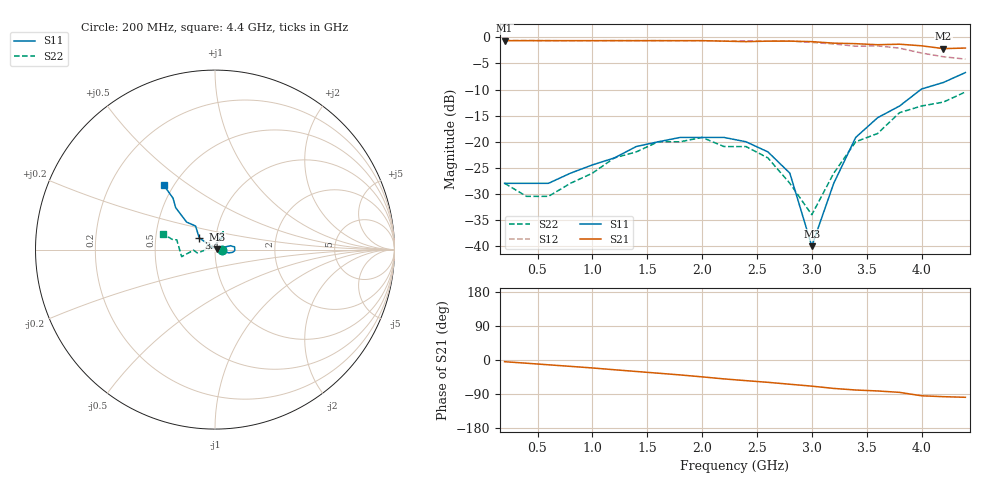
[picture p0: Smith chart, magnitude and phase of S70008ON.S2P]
!  MGS-70008 S PARAMETERS
!  "on" port  LAST UPDATED 07-22-92
# ghz s ma r 50
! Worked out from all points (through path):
!   22 points, 200 MHz to 4.4 GHz, reference 50 ohm
!   highest |S21| = -0.63 dB at 200 MHz (marker M1); lowest = -2.2 dB at 4.2 GHz (marker M2)
!   group delay of S21, straight-line fit = 64.8 ps
!   lowest |S11| = -40.0 dB at 3 GHz (marker M3), VSWR 1.02, Z = 51 + j0.131 ohm
!   |S11| at or under -10 dB: start of sweep to 3.994 GHz
!   |S22| runs from -34.0 to -10.5 dB; largest |S21 - S12| = 0.18
!   S11 on the Smith chart (normalised r, x): 200 MHz: 1.08, -0.01; 3.4 GHz: 0.83, +0.11; 4.4 GHz: 0.44, +0.40
0.2  0.04 -6.2  0.93 -4.5  0.934 -4.4  0.04 -2.5
0.4  0.04 0.3  0.93 -8.5  0.934 -8.3  0.03 10.6
0.6  0.04 7.6  0.93 -12.7  0.93 -12.4  0.03 30.7
0.8  0.05 13.6  0.93 -16.8  0.927 -16.3  0.04 52.8
1  0.06 14.7  0.93 -21.0  0.927 -20.4  0.05 63.0
1.2  0.07 14.5  0.93 -25.7  0.931 -24.5  0.07 67.1
1.4  0.09 14.0  0.93 -30.3  0.93 -28.7  0.08 69.1
1.6  0.1 10.2  0.93 -34.8  0.93 -32.9  0.1 69.2
1.8  0.11 8.1  0.93 -39.4  0.928 -37.6  0.1 66.6
2  0.11 1.4  0.93 -44.5  0.928 -41.8  0.11 65.2
2.2  0.11 -3.2  0.92 -49.9  0.922 -46.8  0.09 62.2
2.4  0.1 -8.5  0.91 -54.5  0.927 -51.5  0.09 60.8
2.6  0.08 -13.1  0.92 -58.9  0.92 -56.2  0.07 60.0
2.8  0.05 -14.1  0.92 -64.0  0.922 -62.4  0.04 70.8
3  0.01 7.4  0.91 -69.0  0.894 -68.7  0.02 127.9
3.2  0.04 141.4  0.88 -75.0  0.864 -74.4  0.05 -178.2
3.4  0.11 143.2  0.87 -79.2  0.823 -79.9  0.1 -169.4
3.6  0.17 129.5  0.85 -81.7  0.828 -85.7  0.12 -178.5
3.8  0.22 135.9  0.86 -85.4  0.788 -91.8  0.19 -168.0
4  0.32 133.2  0.83 -94.4  0.708 -95.0  0.22 165.6
4.2  0.37 129.2  0.78 -96.8  0.652 -99.2  0.24 166.9
4.4  0.46 128.5  0.79 -98.4  0.619 -102.5  0.3 163.4
